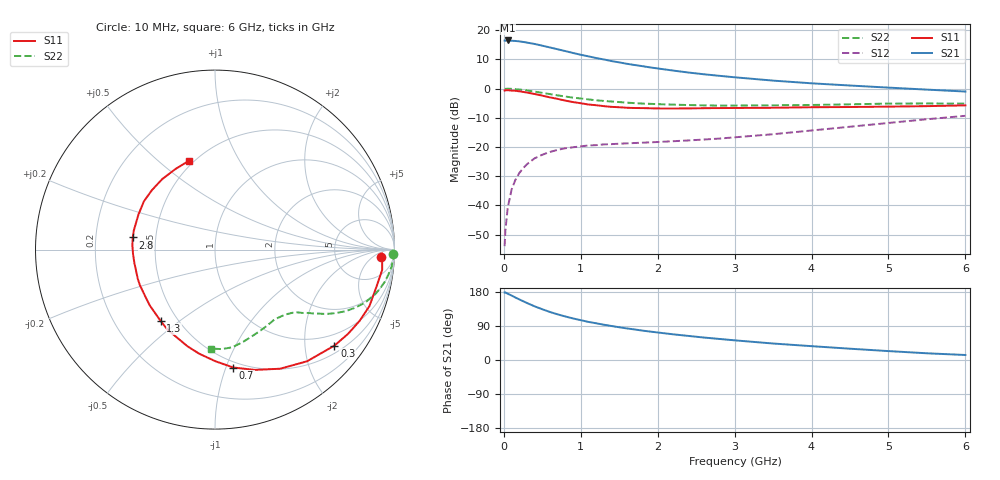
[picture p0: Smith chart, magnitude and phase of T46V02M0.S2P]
! Infineon Technologies  Discrete & RF Semiconductors
! BFR182T
! Si NPN RF Bipolar Junction Transistor in SC75
! VCE = 6 V  IC = 2 mA
! Common Emitter S-Parameters:  October  1999
# GHz  S  MA  R  50
!  f  S11  S21  S12  S22
! GHz  MAG  ANG  MAG  ANG  MAG  ANG  MAG  ANG
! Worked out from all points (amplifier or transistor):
!   36 points, 10 MHz to 6 GHz, reference 50 ohm
!   highest |S21| = 16.5 dB at 50 MHz (marker M1)
!   |S21| within 3 dB of that: start of sweep to 695.8 MHz
!   unconditionally stable (mu >= 1): 2.042 GHz to 4.376 GHz
!   at 250 MHz: K = 0.15, MSG = 21.7 dB, |S12| = -27.3 dB
!   at 1.4 GHz: K = 0.76, MSG = 14.2 dB, |S12| = -19.0 dB
!   at 6 GHz: K = 0.82, MSG = 4.2 dB, |S12| = -9.3 dB
!   lowest NFmin = 1.10 dB at 450 MHz
!   S11 on the Smith chart (normalised r, x): 10 MHz: 20, -11; 300 MHz: 0.68, -2.69; 700 MHz: 0.45, -1.06; 1.3 GHz: 0.40, -0.43; 2.8 GHz: 0.37, +0.06; 6 GHz: 0.47, +0.63
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0.01  0.9249 -2.4  6.639 178.3  0.002 86.0  0.9895 -1.3
0.02  0.9313 -1.3  6.595 178.3  0.0037 92.2  0.987 -1.1
0.05  0.9383 -6.9  6.663 174.9  0.009 89.8  0.9931 -2.8
0.1  0.9232 -12.9  6.586 170.2  0.0185 83.6  0.9887 -5.5
0.15  0.9163 -20.1  6.535 164.9  0.0273 78.7  0.976 -8.2
0.25  0.8772 -32.4  6.29 155.2  0.043 71.6  0.9461 -13.1
0.3  0.8538 -38.8  6.128 150.5  0.0506 69.2  0.928 -15.4
0.4  0.8064 -50.5  5.803 141.6  0.0639 63.2  0.8865 -19.5
0.5  0.7566 -61.3  5.423 133.9  0.0736 58.6  0.8441 -22.6
0.6  0.706 -71.7  5.052 126.7  0.0822 54.2  0.8038 -25.3
0.7  0.6647 -81.2  4.703 120.4  0.0892 51.3  0.7641 -27.5
0.9  0.5868 -98.6  4.065 109.6  0.0988 45.9  0.699 -30.8
1.1  0.533 -113.7  3.559 100.5  0.106 43.3  0.6513 -33.1
1.3  0.4997 -127.3  3.15 93.1  0.1107 41.7  0.6135 -35.1
1.5  0.4787 -139.2  2.807 86.4  0.1136 41.2  0.5873 -36.7
1.8  0.4628 -155.1  2.42 77.6  0.1183 41.8  0.5536 -39.6
2.2  0.4554 -170.6  2.034 67.8  0.1254 44.3  0.5309 -43.3
2.8  0.4632 171.6  1.653 55.6  0.1391 49.2  0.511 -50.5
3.5  0.4692 155.3  1.368 43.5  0.1653 54.9  0.516 -59.1
4.5  0.483 136.6  1.127 29.8  0.222 58.5  0.5369 -72.9
5.5  0.4999 116.3  0.959 17.7  0.2983 57.0  0.5556 -86.3
6  0.5155 106.6  0.889 13.2  0.3413 54.3  0.5515 -92.4
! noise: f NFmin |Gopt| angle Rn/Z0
0.45  1.1  0.42  29  0.36
0.9  1.2  0.4  58  0.3
1.8  1.85  0.32  126  0.22
